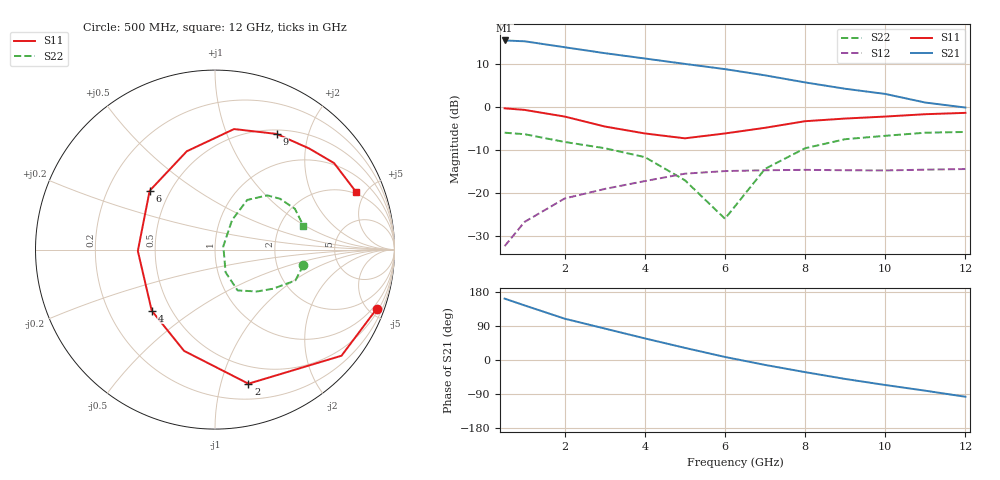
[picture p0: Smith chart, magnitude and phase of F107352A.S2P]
!!ATF-10735
!S-PARAMETERS at Vds=2V  Id=25mA.  LAST UPDATED 07-22-92
# ghz s ma r 50
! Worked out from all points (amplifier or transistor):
!   13 points, 500 MHz to 12 GHz, reference 50 ohm
!   highest |S21| = 15.4 dB at 500 MHz (marker M1)
!   |S21| within 3 dB of that: start of sweep to 3.039 GHz
!   unconditionally stable (mu >= 1): 4.871 GHz to end of sweep
!   at 2 GHz: K = 0.61, MSG = 17.6 dB, |S12| = -21.3 dB
!   at 6 GHz: K = 1.04, MAG = 10.6 dB, |S12| = -14.9 dB
!   at 12 GHz: K = 1.03, MAG = 6.2 dB, |S12| = -14.5 dB
!   lowest NFmin = 0.70 dB at 500 MHz
!   S11 on the Smith chart (normalised r, x): 500 MHz: 0.67, -5.59; 2 GHz: 0.33, -1.22; 4 GHz: 0.39, -0.35; 6 GHz: 0.39, +0.33; 9 GHz: 0.55, +1.52; 12 GHz: 1.90, +4.35
0.5  0.96 -20.0  5.9 162.0  0.024 77.0  0.5 -10.0
1  0.92 -40.0  5.77 144.0  0.046 66.0  0.48 -21.0
2  0.77 -76.0  4.92 109.0  0.086 52.0  0.39 -34.0
3  0.59 -107.0  4.2 83.0  0.111 40.0  0.33 -45.0
4  0.49 -136.0  3.64 57.0  0.137 24.0  0.26 -61.0
5  0.43 -179.0  3.15 32.0  0.167 9.0  0.14 -65.0
6  0.49 138.0  2.74 8.0  0.179 -5.0  0.05 22.0
7  0.57 106.0  2.32 -13.0  0.183 -18.0  0.19 60.0
8  0.68 81.0  1.92 -32.0  0.185 -33.0  0.33 57.0
9  0.73 62.0  1.62 -50.0  0.183 -40.0  0.42 46.0
10  0.77 47.0  1.41 -66.0  0.182 -52.0  0.46 38.0
11  0.82 36.0  1.12 -81.0  0.186 -67.0  0.5 27.0
12  0.85 22.0  0.98 -97.0  0.189 -75.0  0.51 15.0
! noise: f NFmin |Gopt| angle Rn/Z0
0.5  0.7  0.94  19  0.65
1  0.8  0.88  41  0.52
2  0.9  0.75  85  0.27
4  1.2  0.48  159  0.08
6  1.4  0.46  -122  0.08
8  1.7  0.53  -71  0.43
12  2  0.69  -14  1.04
